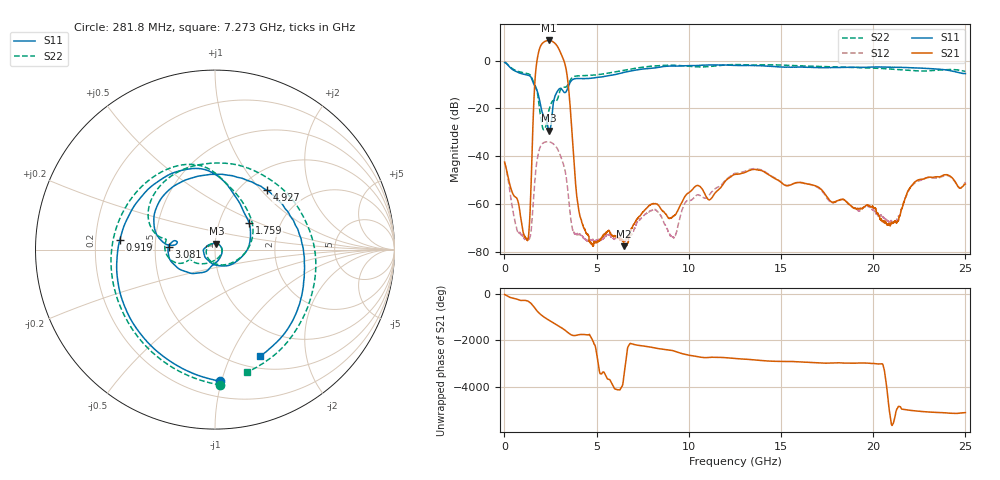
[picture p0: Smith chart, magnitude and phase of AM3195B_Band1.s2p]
!Agilent Technologies,E8364B,MY43040894,A.07.50.67
!Agilent E8364B: A.07.50.67
!Date: Wednesday, July 07, 2021 13:16:15
!Correction: S11(Full 2 Port(1,2))
!S21(Full 2 Port(1,2))
!S12(Full 2 Port(1,2))
!S22(Full 2 Port(1,2))
!S2P File: Measurements: S11, S21, S12, S22:
# Hz S  dB  R 50
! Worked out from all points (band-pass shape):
!   8001 points, 10 MHz to 25 GHz, reference 50 ohm
!   highest |S21| = 8.38 dB at 2.412 GHz (marker M1); lowest = -77.5 dB at 6.492 GHz (marker M2)
!   |S21| within 3 dB of the highest: 1.924 GHz to 2.914 GHz (990.5 MHz wide, 40.9 % of centre)
!   lowest |S11| = -29.2 dB at 2.415 GHz (marker M3), VSWR 1.07, Z = 50.7 + j3.41 ohm
!   |S11| at or under -10 dB: 1.605 GHz to 3.507 GHz (1.902 GHz wide, 74.4 % of centre)
!   |S22| runs from -28.9 to -0.6 dB; largest |S21 - S12| = 2.6
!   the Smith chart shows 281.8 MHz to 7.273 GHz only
!   S11 on the Smith chart (normalised r, x): 281.8 MHz: 0.31, -0.99; 919 MHz: 0.31, +0.04; 1.759 GHz: 1.39, +0.43; 3.081 GHz: 0.59, +0.02; 4.927 GHz: 1.32, +1.08; 7.273 GHz: 0.64, -1.30
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1e7  -0.83 -15.9  -42.38 -36.7  -42.72 -37.2  -0.62 -16.9
2.817662e8  -2.69 -87.9  -51.41 -152.6  -53.85 -150.8  -2.44 -87.7
9.190112e8  -5.46 174.4  -67.42 70.0  -72.65 25.1  -4.88 174.3
1.30948e9  -6.19 122.6  -73.17 21.8  -74.74 97.5  -5.59 124.4
1.7593e9  -12.37 37.6  -0.37 -13.6  -42.17 176.1  -12.36 28.7
1.987334e9  -19.78 -62.6  6.45 170.5  -35.35 1.2  -24.63 -137.8
2.143521e9  -23.13 -135.7  7.74 76.9  -34.20 -90.8  -28.82 57.6
2.280966e9  -24.06 177.8  8.24 4.7  -33.91 -162.3  -26.23 -67.4
2.412164e9  -29.23 79.4  8.38 -59.8  -33.92 133.5  -20.82 -122.5
2.415288e9  -29.23 76.2  8.38 -61.3  -33.93 132.0  -20.73 -123.1
2.65894e9  -17.34 -114.2  7.70 -177.2  -34.82 17.1  -16.67 -161.2
2.846365e9  -13.15 -148.9  6.23 93.6  -36.48 -70.3  -16.58 -160.7
3.080646e9  -11.71 176.3  2.65 -20.0  -40.59 179.5  -11.53 -171.3
4.177082e9  -7.56 100.1  -66.84 45.1  -72.96 161.8  -6.36 99.1
4.926782e9  -7.13 48.6  -75.99 -91.8  -75.37 -11.1  -6.01 47.3
6.491781e9  -4.94 -35.4  -77.48 147.2  -74.94 -113.4  -4.07 -40.3
7.272719e9  -3.80 -67.1  -65.36 -61.8  -67.04 -80.8  -3.02 -75.5
8.341041e9  -2.87 -105.1  -60.34 159.2  -63.34 149.7  -2.17 -117.0
1.2505e10  -2.02 140.0  -47.53 92.4  -47.05 91.9  -1.68 126.2
1.667208e10  -2.86 19.5  -51.86 -77.4  -52.04 -80.1  -2.37 3.3
2.083604e10  -2.81 -69.5  -68.19 -73.7  -67.16 -79.1  -3.49 -82.1
2.5e10  -5.44 -124.4  -51.54 -76.2  -50.67 -76.2  -4.52 -132.5
